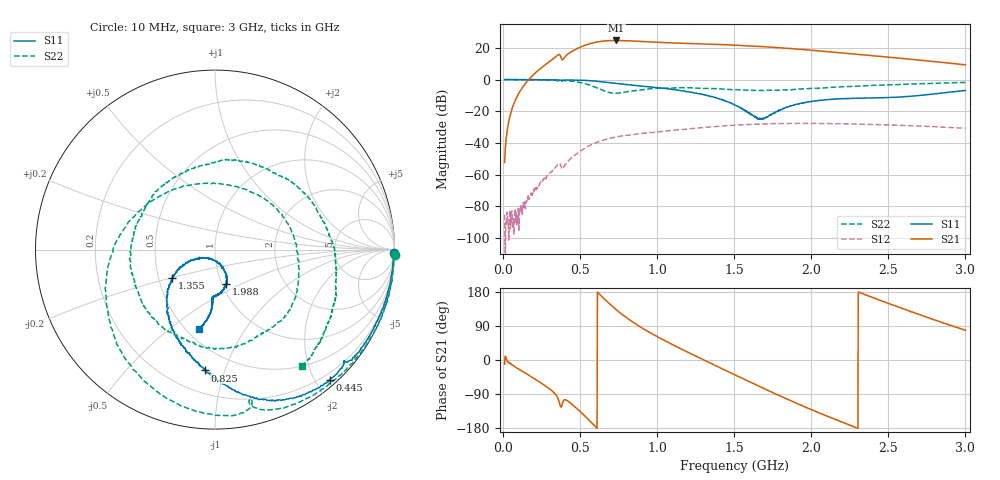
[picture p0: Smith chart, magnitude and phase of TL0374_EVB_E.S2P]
!Agilent Technologies,E5071C,MY46523237,B.13.01
!Date: Thu Sep 16 14:19:08 2021
!Data & Calibration Information:
!Freq	S11:SOLT2(ON)	S21:SOLT2(ON)	S12:SOLT2(ON)	S22:SOLT2(ON)
!PortZ  Port1:50+j0  Port2:50+j0
!Above PortZ is port z conversion or system Z0 setting when saving the data.
!When reading, reference impedance value at option line is always used.
# Hz S dB R 50
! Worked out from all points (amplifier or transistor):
!   1197 points, 10 MHz to 3 GHz, reference 50 ohm
!   highest |S21| = 24.7 dB at 735 MHz (marker M1)
!   |S21| within 3 dB of that: 533.1 MHz to 1.514 GHz (980.9 MHz wide, 95.8 % of centre)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
!   unconditionally stable (mu >= 1): 10.65 MHz to 53.22 MHz; 145.8 MHz to 466.5 MHz; 600.7 MHz to end of sweep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
!   at 507.5 MHz: K = 1.01, MAG = 32.1 dB, |S12| = -44.8 dB
!   at 1.505 GHz: K = 1.12, MAG = 23.2 dB, |S12| = -28.8 dB
!   at 3 GHz: K = 1.45, MAG = 16.1 dB, |S12| = -30.8 dB
!   S11 on the Smith chart (normalised r, x): 10 MHz: open; 445 MHz: 0.09, -2.21; 825 MHz: 0.35, -0.86; 1.355 GHz: 0.59, -0.20; 1.988 GHz: 1.05, -0.41; 3 GHz: 0.57, -0.64
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1e7  -0.01 -1.1  -52.37 -11.1  -85.41 157.5  0.02 -1.6
1.65e8  -0.07 -17.4  -0.14 -39.9  -73.67 -154.7  -0.03 -30.1
2.875e8  -0.13 -30.7  10.37 -72.0  -60.96 -164.8  -0.22 -57.0
3.55e8  -0.17 -38.9  15.51 -100.5  -53.66 178.2  -0.80 -75.4
3.875e8  -0.40 -41.2  12.55 -111.1  -56.47 168.3  -0.79 -78.9
4.45e8  -0.27 -48.7  17.70 -116.1  -49.36 173.9  -0.99 -101.1
5.1e8  -0.45 -57.5  20.86 -139.6  -44.69 156.1  -2.06 -129.0
5.625e8  -0.70 -64.8  22.63 -160.9  -41.75 139.8  -3.57 -156.1
6.275e8  -1.24 -74.0  24.01 172.7  -39.05 118.3  -5.91 162.3
6.75e8  -1.78 -79.7  24.53 154.0  -37.54 102.3  -7.76 126.6
7.35e8  -2.47 -86.0  24.72 132.6  -36.20 84.6  -8.69 77.2
8.25e8  -3.41 -94.6  24.46 104.8  -35.00 61.6  -7.40 22.6
1.0075e9  -5.18 -110.9  23.52 60.0  -33.04 24.9  -5.42 -41.5
1.1775e9  -7.30 -128.2  22.92 24.7  -31.40 -4.7  -5.14 -84.2
1.355e9  -10.81 -146.3  22.30 -10.0  -29.85 -34.7  -5.67 -127.2
1.505e9  -16.25 -155.8  21.79 -39.2  -28.85 -60.5  -6.40 -166.3
1.7225e9  -23.00 -80.1  20.59 -80.8  -27.96 -98.0  -6.71 133.2
1.9875e9  -14.05 -72.1  18.65 -128.7  -27.69 -141.1  -5.72 69.6
2.005e9  -13.82 -72.7  18.45 -131.8  -27.71 -143.9  -5.59 65.7
2.2075e9  -12.10 -85.1  16.76 -164.7  -27.96 -174.6  -4.51 29.8
2.5025e9  -11.35 -92.7  14.14 149.0  -28.68 143.4  -3.32 -8.1
3e9  -6.87 -101.4  9.29 78.7  -30.83 78.3  -1.85 -53.1
